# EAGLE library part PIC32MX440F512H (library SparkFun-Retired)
PIC32MX440F512H Retired: IC-09313
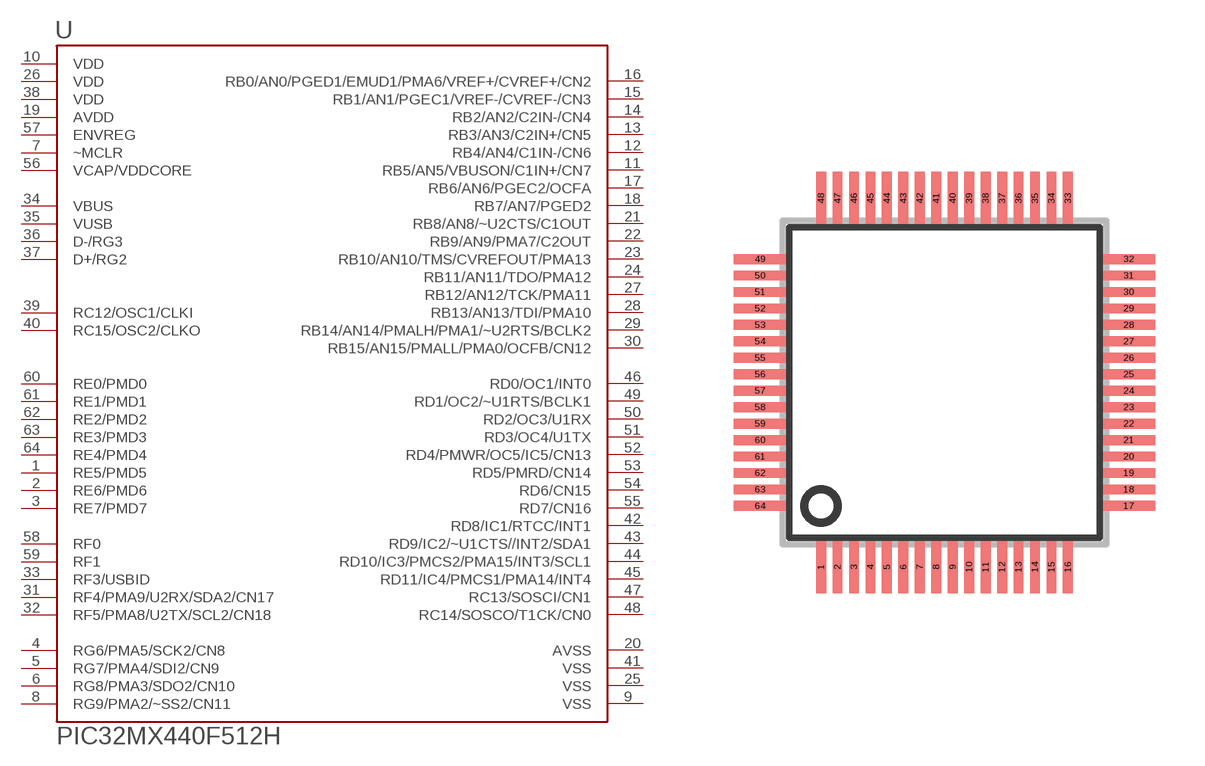
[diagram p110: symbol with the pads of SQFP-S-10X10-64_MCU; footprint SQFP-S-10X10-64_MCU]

Designator prefix -

## PIC32MX440F512H  [SQFP-S-10X10-64_MCU]
1  RE5/PMD5
2  RE6/PMD6
3  RE7/PMD7
4  RG6/PMA5/SCK2/CN8
5  RG7/PMA4/SDI2/CN9
6  RG8/PMA3/SDO2/CN10
7  ~MCLR
8  RG9/PMA2/~SS2/CN11
9  VSS
10  VDD
11  RB5/AN5/VBUSON/C1IN+/CN7
12  RB4/AN4/C1IN-/CN6
13  RB3/AN3/C2IN+/CN5
14  RB2/AN2/C2IN-/CN4
15  RB1/AN1/PGEC1/VREF-/CVREF-/CN3
16  RB0/AN0/PGED1/EMUD1/PMA6/VREF+/CVREF+/CN2
17  RB6/AN6/PGEC2/OCFA
18  RB7/AN7/PGED2
19  AVDD
20  AVSS
21  RB8/AN8/~U2CTS/C1OUT
22  RB9/AN9/PMA7/C2OUT
23  RB10/AN10/TMS/CVREFOUT/PMA13
24  RB11/AN11/TDO/PMA12
25  VSS
26  VDD
27  RB12/AN12/TCK/PMA11
28  RB13/AN13/TDI/PMA10
29  RB14/AN14/PMALH/PMA1/~U2RTS/BCLK2
30  RB15/AN15/PMALL/PMA0/OCFB/CN12
31  RF4/PMA9/U2RX/SDA2/CN17
32  RF5/PMA8/U2TX/SCL2/CN18
33  RF3/USBID
34  VBUS
35  VUSB
36  D-/RG3
37  D+/RG2
38  VDD
39  RC12/OSC1/CLKI
40  RC15/OSC2/CLKO
41  VSS
42  RD8/IC1/RTCC/INT1
43  RD9/IC2/~U1CTS//INT2/SDA1
44  RD10/IC3/PMCS2/PMA15/INT3/SCL1
45  RD11/IC4/PMCS1/PMA14/INT4
46  RD0/OC1/INT0
47  RC13/SOSCI/CN1
48  RC14/SOSCO/T1CK/CN0
49  RD1/OC2/~U1RTS/BCLK1
50  RD2/OC3/U1RX
51  RD3/OC4/U1TX
52  RD4/PMWR/OC5/IC5/CN13
53  RD5/PMRD/CN14
54  RD6/CN15
55  RD7/CN16
56  VCAP/VDDCORE
57  ENVREG
58  RF0
59  RF1
60  RE0/PMD0
61  RE1/PMD1
62  RE2/PMD2
63  RE3/PMD3
64  RE4/PMD4

## Footprint SQFP-S-10X10-64_MCU (pad centres in mm)
QFP64 shrink quad flat pack, square
smd 0.3 x 1.6: 1 -3.75,-5.6; 2 -3.25,-5.6; 3 -2.75,-5.6; 4 -2.25,-5.6; 5 -1.75,-5.6; 6 -1.25,-5.6; 7 -0.75,-5.6; 8 -0.25,-5.6; 9 0.25,-5.6; 10 0.75,-5.6; 11 1.25,-5.6; 12 1.75,-5.6; 13 2.25,-5.6; 14 2.75,-5.6; 15 3.25,-5.6; 16 3.75,-5.6; 33 3.75,5.6; 34 3.25,5.6; 35 2.75,5.6; 36 2.25,5.6; 37 1.75,5.6; 38 1.25,5.6; 39 0.75,5.6; 40 0.25,5.6; 41 -0.25,5.6; 42 -0.75,5.6; 43 -1.25,5.6; 44 -1.75,5.6; 45 -2.25,5.6; 46 -2.75,5.6; 47 -3.25,5.6; 48 -3.75,5.6
smd 1.6 x 0.3: 17 5.6,-3.75; 18 5.6,-3.25; 19 5.6,-2.75; 20 5.6,-2.25; 21 5.6,-1.75; 22 5.6,-1.25; 23 5.6,-0.75; 24 5.6,-0.25; 25 5.6,0.25; 26 5.6,0.75; 27 5.6,1.25; 28 5.6,1.75; 29 5.6,2.25; 30 5.6,2.75; 31 5.6,3.25; 32 5.6,3.75; 49 -5.6,3.75; 50 -5.6,3.25; 51 -5.6,2.75; 52 -5.6,2.25; 53 -5.6,1.75; 54 -5.6,1.25; 55 -5.6,0.75; 56 -5.6,0.25; 57 -5.6,-0.25; 58 -5.6,-0.75; 59 -5.6,-1.25; 60 -5.6,-1.75; 61 -5.6,-2.25; 62 -5.6,-2.75; 63 -5.6,-3.25; 64 -5.6,-3.75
